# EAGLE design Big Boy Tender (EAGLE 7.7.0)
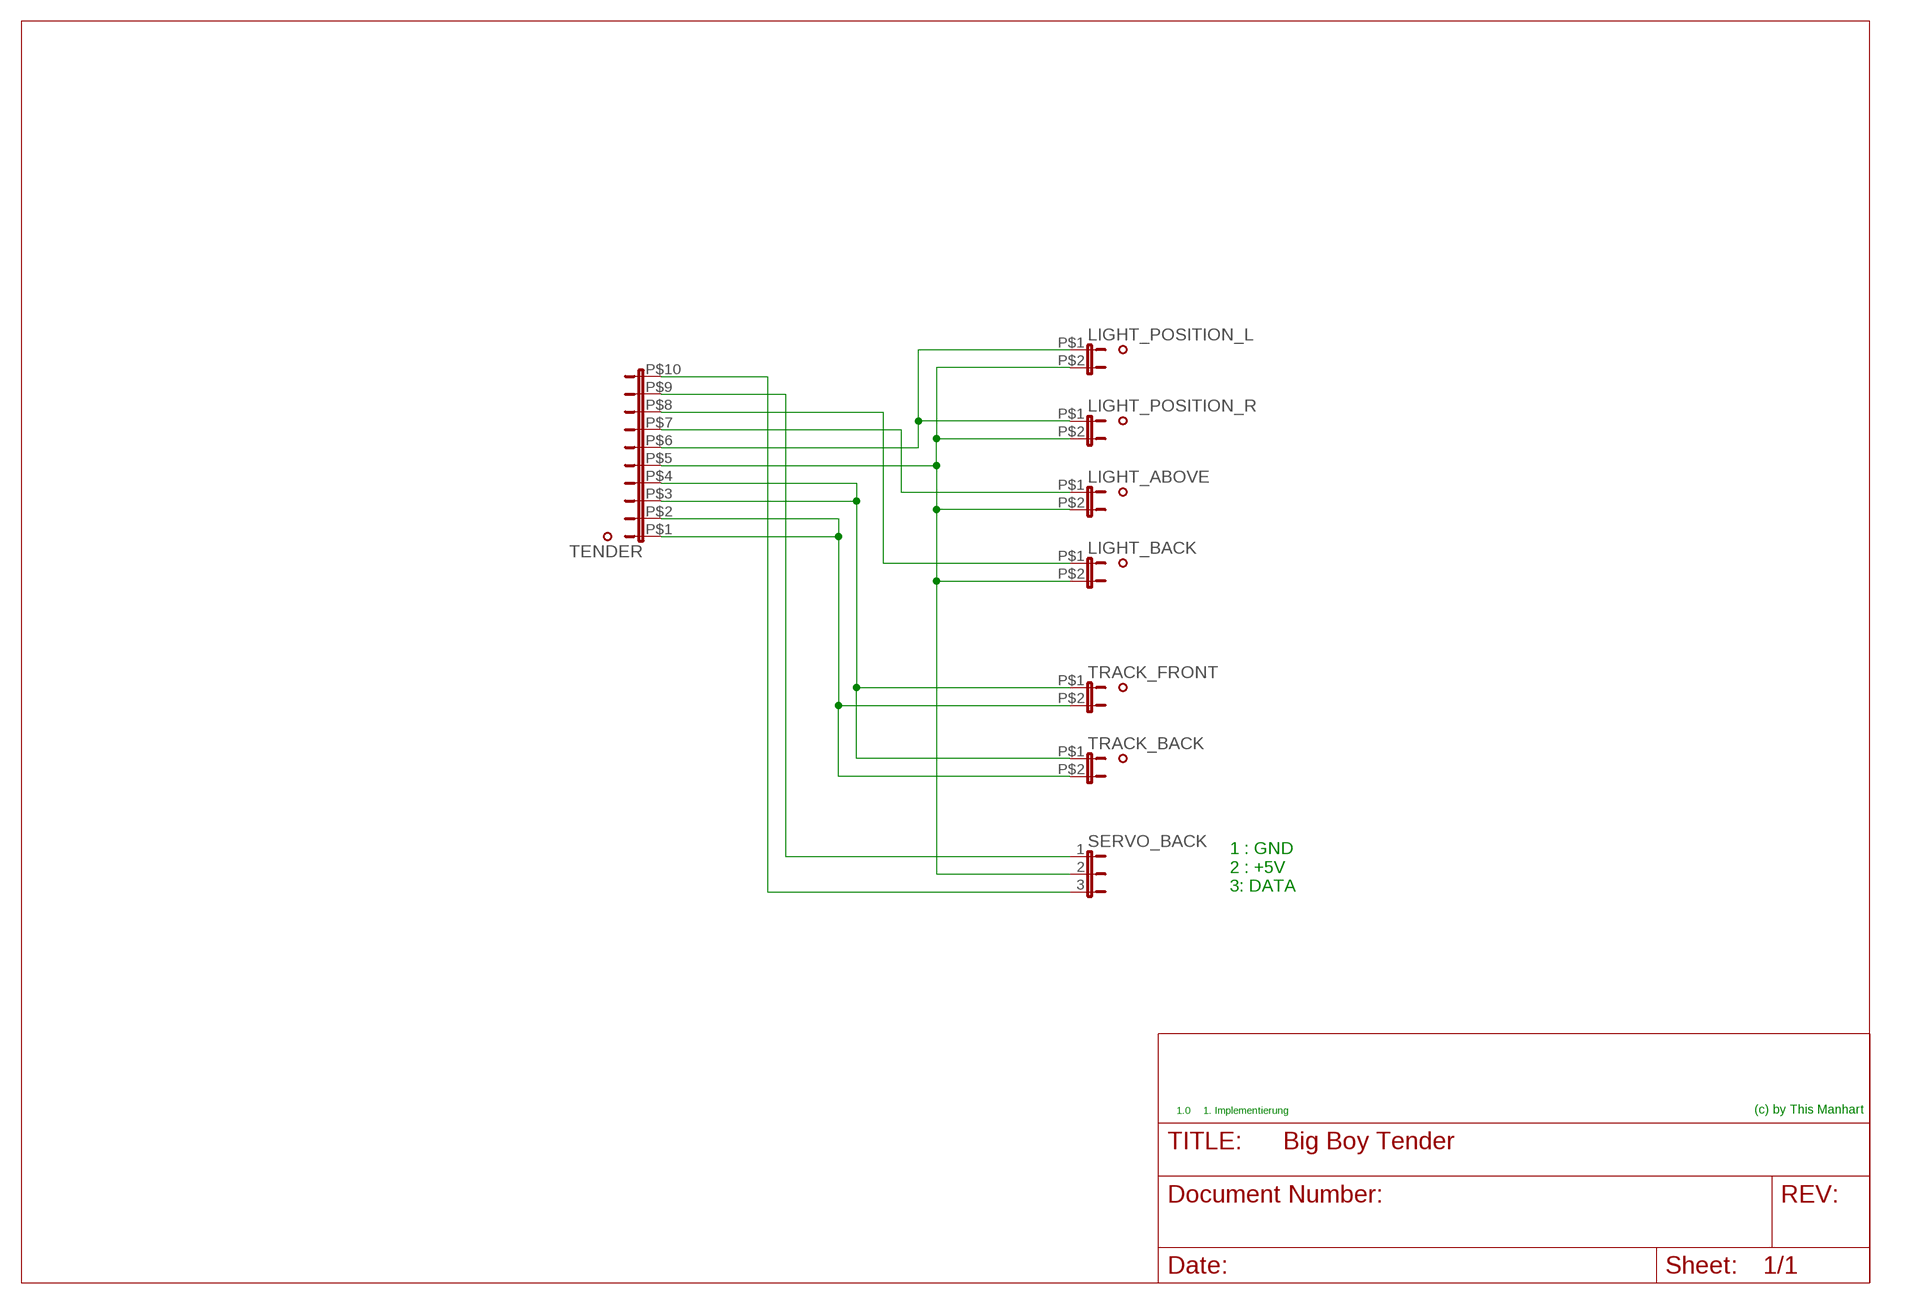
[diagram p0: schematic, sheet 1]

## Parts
LIGHT_ABOVE  DUBOX_2POL90  [DUBOX_2POL_STIFTLEISTE_90]
LIGHT_BACK  DUBOX_2POL90  [DUBOX_2POL_STIFTLEISTE_90]
LIGHT_POSITION_L  DUBOX_2POL90  [DUBOX_2POL_STIFTLEISTE_90]
LIGHT_POSITION_R  DUBOX_2POL90  [DUBOX_2POL_STIFTLEISTE_90]
SERVO_BACK  JUMPER_3PDIP  [JUMPER_3P_2.54]
TENDER  DUBOX_10POL2R_90  [DUBOX_10POL_STIFTLEISTE_90_2R]
TRACK_BACK  DUBOX_2POL90  [DUBOX_2POL_STIFTLEISTE_90]
TRACK_FRONT  DUBOX_2POL90  [DUBOX_2POL_STIFTLEISTE_90]

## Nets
N$1: TENDER.P$1 TENDER.P$2 TRACK_BACK.P$2 TRACK_FRONT.P$2
N$2: TENDER.P$3 TENDER.P$4 TRACK_BACK.P$1 TRACK_FRONT.P$1
N$3: LIGHT_ABOVE.P$2 LIGHT_BACK.P$2 LIGHT_POSITION_L.P$2 LIGHT_POSITION_R.P$2 SERVO_BACK.2 TENDER.P$5
N$4: LIGHT_POSITION_L.P$1 LIGHT_POSITION_R.P$1 TENDER.P$6
N$5: LIGHT_ABOVE.P$1 TENDER.P$7
N$6: LIGHT_BACK.P$1 TENDER.P$8
N$7: SERVO_BACK.1 TENDER.P$9
N$8: SERVO_BACK.3 TENDER.P$10

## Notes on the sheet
- 1 : GND
  2 : +5V
  3: DATA
- 1.0 | 1. Implementierung | (c) by This Manhart

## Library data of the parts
LIGHT_ABOVE LIGHT_BACK LIGHT_POSITION_L LIGHT_POSITION_R TRACK_BACK TRACK_FRONT = 0_mm:DUBOX_2POL: DUBOX 2pol Buchse
SERVO_BACK = 0_mm:JUMPER_3P
TENDER = 0_mm:DUBOX_10POL

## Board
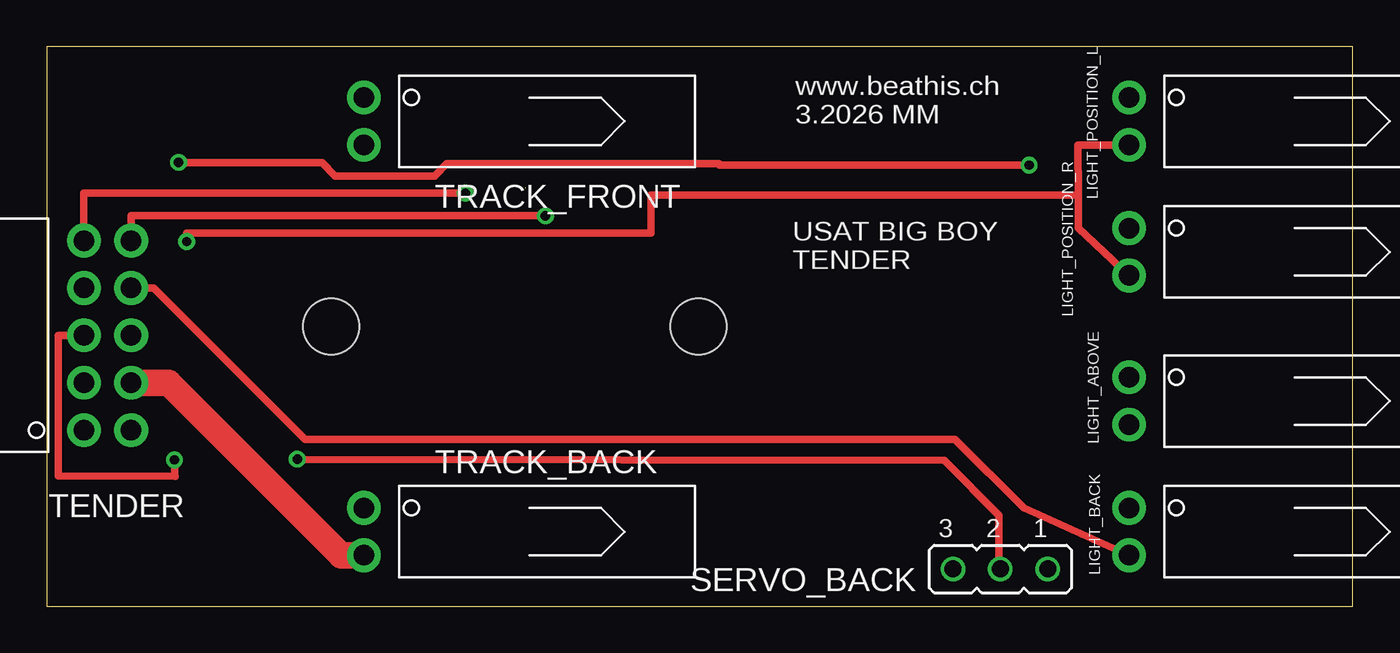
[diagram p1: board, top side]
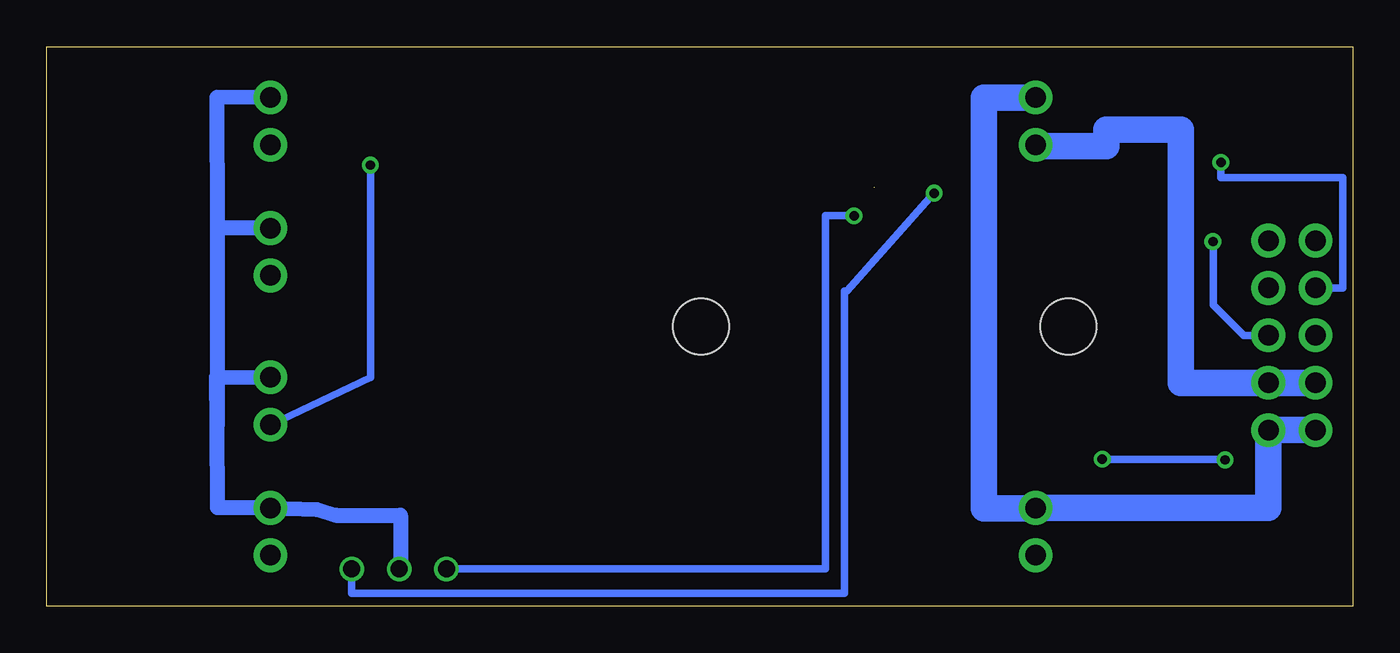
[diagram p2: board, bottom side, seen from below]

Size 70 x 30 mm. Coordinates in mm from the lower left corner, seen from the top.
Outline: 25.65,22.45 25.66,22.45
Outline: 70,0 70,30 0,30 0,0 70,0
Copper layers (1*16): Top 0.035mm / dielectric 1.5mm / Bottom 0.035mm
Design rules "PCB-POOL Standard": minimum track width 0.15mm, minimum drill 0.3mm, track to track 0.15mm, track to pad 0.15mm, pad to pad 0.15mm, via to via 0.15mm, smd to smd 0.15mm, copper to edge 0.3mm, drill to drill 0.2mm, minimum pad ring 0.2mm, minimum via ring 0.15mm, stop-mask expansion 0.075mm, vias tented up to drill 0mil, thermal gap 0.2mm
Holes 3 mm at 34.94,15 15.24,15

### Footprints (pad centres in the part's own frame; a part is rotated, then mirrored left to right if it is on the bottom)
DUBOX_2POL_STIFTLEISTE_90 = drill 1.1 pad 1.8: P$1 1.27,0; P$2 -1.27,0
JUMPER_3P_2.54 = drill 0.914: 1 -2.54,0; 2 0,0; 3 2.54,0
DUBOX_10POL_STIFTLEISTE_90_2R = drill 1.1 pad 1.8: P$1 -1.27,0; P$2 -1.27,-2.54; P$3 1.27,0; P$4 1.27,-2.54; P$5 3.81,0; P$6 3.81,-2.54; P$7 6.35,0; P$8 6.35,-2.54; P$9 8.89,0; P$10 8.89,-2.54

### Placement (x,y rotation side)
LIGHT_ABOVE  58,11 270 top
LIGHT_BACK  58,4 270 top
LIGHT_POSITION_L  58,26 270 top
LIGHT_POSITION_R  58,19 270 top
SERVO_BACK  51.11,2 180 top
TENDER  1.99,10.71 90 top
TRACK_BACK  17,4 270 top
TRACK_FRONT  17,26 270 top

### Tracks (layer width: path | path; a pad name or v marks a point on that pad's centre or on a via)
N$1
  Bottom 1.422: TENDER.P$1 TENDER.P$2 4.53,5.27 TRACK_BACK.P$2 17,5.24 19.78,5.24 19.78,27.27 TRACK_FRONT.P$2
N$2
  Top 1.422: TRACK_BACK.P$1 15.78,2.73 6.53,11.98 TENDER.P$4
  Bottom 1.422: TENDER.P$3 TENDER.P$4 9.22,11.98 9.22,25.55 13.2,25.55 13.2,24.67 17,24.67 TRACK_FRONT.P$1
N$3  (via drill 0.5 pad 0.81)
  Top 0.406: v13.43,7.88 48.1,7.82 51.04,4.88 51.04,2.07 SERVO_BACK.2 | TENDER.P$5 0.63,14.52 0.63,7 6.89,6.95 6.85,6.99 v6.85,7.84
  Bottom 0.406: v13.43,7.88 6.89,7.88 v6.85,7.84
  Bottom 0.813: 60.85,9.72 60.87,9.75 60.84,5.28 LIGHT_BACK.P$2 55.51,5.19 54.51,4.88 51.04,4.88 51.04,2.07 SERVO_BACK.2 | 60.85,9.72 60.9,12.29 LIGHT_ABOVE.P$2 | LIGHT_POSITION_R.P$2 60.85,20.27 | 60.85,20.27 60.85,9.72 | LIGHT_POSITION_L.P$2 60.88,27.28 60.85,20.27
N$4  (via drill 0.5 pad 0.81)
  Top 0.406: v7.5,19.55 7.5,20.01 32.4,20.01 32.4,22.03 55.3,22.03 | 55.3,22.03 55.27,24.72 LIGHT_POSITION_L.P$1 | LIGHT_POSITION_R.P$1 55.3,20.27 55.3,22.03
  Bottom 0.406: TENDER.P$6 5.85,14.52 7.47,16.14 7.47,19.52 v7.5,19.55
N$5  (via drill 0.5 pad 0.81)
  Top 0.406: v7.07,23.79 14.75,23.79 15.47,23.07 20.79,23.07 21.44,23.72 36.03,23.72 36.06,23.69 36.06,23.65 v52.65,23.65
  Bottom 0.406: TENDER.P$7 0.55,17.06 0.55,22.97 7.07,22.97 v7.07,23.79 | LIGHT_ABOVE.P$1 52.65,12.27 v52.65,23.65
N$6
  Top 0.406: LIGHT_BACK.P$1 52.36,5.27 48.68,8.95 13.85,8.95 5.74,17.06 TENDER.P$8
N$7  (via drill 0.5 pad 0.81)
  Top 0.406: v22.44,22.14 1.99,22.14 TENDER.P$9
  Bottom 0.406: SERVO_BACK.1 53.65,0.7 27.25,0.7 27.25,16.89 27.12,16.89 v22.44,22.14
N$8  (via drill 0.5 pad 0.81)
  Top 0.406: v26.73,20.93 4.53,20.93 TENDER.P$10
  Bottom 0.406: SERVO_BACK.3 28.26,2 28.26,20.93 v26.73,20.93

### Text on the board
tNames: www.beathis.ch / 3.2026 MM | USAT BIG BOY / TENDER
